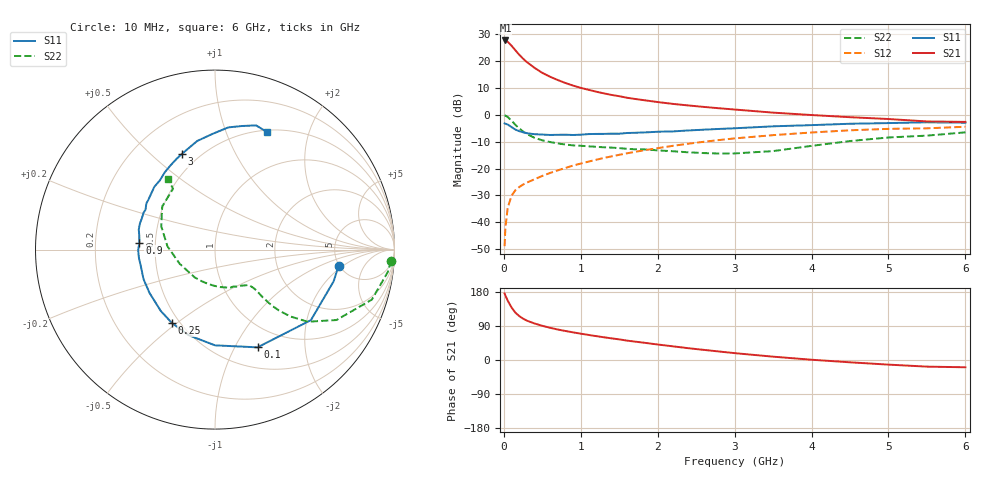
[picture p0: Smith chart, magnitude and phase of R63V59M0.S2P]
! SIEMENS Small Signal Semiconductors
! BFR193
! Si NPN RF Bipolar Junction Transistor in SOT23
! VCE = 3.5 V  IC = 9 mA
! Common Emitter S-Parameters:  May  1996
# GHz  S  MA  R  50
!  f  S11  S21  S12  S22
! GHz  MAG  ANG  MAG  ANG  MAG  ANG  MAG  ANG
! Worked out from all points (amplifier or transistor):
!   36 points, 10 MHz to 6 GHz, reference 50 ohm
!   highest |S21| = 27.7 dB at 20 MHz (marker M1)
!   |S21| within 3 dB of that: start of sweep to 130.5 MHz
!   unconditionally stable (mu >= 1): 758.8 MHz to 1.943 GHz
!   at 250 MHz: K = 0.61, MSG = 23.4 dB, |S12| = -25.9 dB
!   at 1.4 GHz: K = 1.04, MAG = 10.2 dB, |S12| = -15.4 dB
!   at 6 GHz: K = 0.95, MSG = 0.9 dB, |S12| = -4.4 dB
!   S11 on the Smith chart (normalised r, x): 10 MHz: 4.94, -1.71; 100 MHz: 0.74, -1.24; 250 MHz: 0.45, -0.48; 900 MHz: 0.41, +0.04; 3 GHz: 0.40, +0.63; 6 GHz: 0.52, +1.41
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0.01  0.6948 -7.4  24.34 175.3  0.0036 85.2  0.9839 -3.6
0.02  0.6841 -15.0  24.34 170.1  0.0079 80.6  0.9708 -7.4
0.05  0.6634 -36.3  23.03 156.8  0.0185 73.6  0.9172 -17.7
0.1  0.5939 -66.5  19.41 138.7  0.0313 64.0  0.7824 -30.1
0.15  0.5334 -90.0  15.97 124.9  0.0396 57.3  0.6544 -37.9
0.2  0.4992 -107.0  13.21 116.0  0.0454 55.1  0.5606 -41.6
0.25  0.4747 -120.2  11.14 109.1  0.0505 54.0  0.4922 -43.6
0.3  0.4561 -131.5  9.615 103.8  0.055 54.6  0.4409 -44.6
0.4  0.4375 -146.6  7.498 96.3  0.0635 56.4  0.3747 -45.0
0.5  0.4308 -157.6  6.066 90.2  0.0733 57.8  0.336 -44.7
0.6  0.4235 -166.7  5.141 85.1  0.083 59.1  0.3127 -44.7
0.7  0.4263 -173.7  4.468 80.5  0.0927 60.6  0.2951 -45.2
0.9  0.4229 174.8  3.516 72.9  0.1139 61.8  0.271 -46.7
1.1  0.4394 165.2  2.935 66.2  0.135 62.2  0.2604 -49.9
1.3  0.4432 157.0  2.519 60.0  0.158 61.6  0.2495 -53.7
1.6  0.4607 146.1  2.089 51.2  0.1927 60.2  0.2342 -61.6
2.2  0.4933 128.4  1.603 36.0  0.2663 54.8  0.2105 -82.5
3  0.5638 109.2  1.26 18.1  0.3655 44.3  0.1919 -126.2
3.5  0.6133 99.3  1.103 8.8  0.4202 36.7  0.212 -158.1
4.5  0.6848 83.8  0.907 -6.1  0.5169 21.6  0.3262 156.6
5.5  0.729 71.7  0.756 -17.5  0.5631 5.9  0.4116 124.6
6  0.7159 66.0  0.741 -19.2  0.6019 1.2  0.4736 123.6
